(* Logix 5000 DataType export R8AI8DIDO_Seneca_InData; software revision 35.00 *)

TYPE R8AI8DIDO_Seneca_InData :   // User Define Measure Data Type for Seneca R-8AI-8DIDO-2-E Device
STRUCT
   DIN1 : BOOL;
   DIN2 : BOOL;
   DIN3 : BOOL;
   DIN4 : BOOL;
   DIN5 : BOOL;
   DIN6 : BOOL;
   DIN7 : BOOL;
   DIN8 : BOOL;
   COUNT1 : UDINT;
   COUNT2 : UDINT;
   COUNT3 : UDINT;
   COUNT4 : UDINT;
   COUNT5 : UDINT;
   COUNT6 : UDINT;
   COUNT7 : UDINT;
   COUNT8 : UDINT;
   FREQ1 : REAL;
   FREQ2 : REAL;
   FREQ3 : REAL;
   FREQ4 : REAL;
   FREQ5 : REAL;
   FREQ6 : REAL;
   FREQ7 : REAL;
   FREQ8 : REAL;
   AIN1 : REAL;
   AIN2 : REAL;
   AIN3 : REAL;
   AIN4 : REAL;
   AIN5 : REAL;
   AIN6 : REAL;
   AIN7 : REAL;
   AIN8 : REAL;
   FLAGS1 : INT;
   FLAGS2 : INT;
   FLAGS3 : INT;
   CJ1_2 : REAL;
   CJ3_4 : REAL;
   CJ5_6 : REAL;
   CJ7_8 : REAL;
END_STRUCT
END_TYPE
